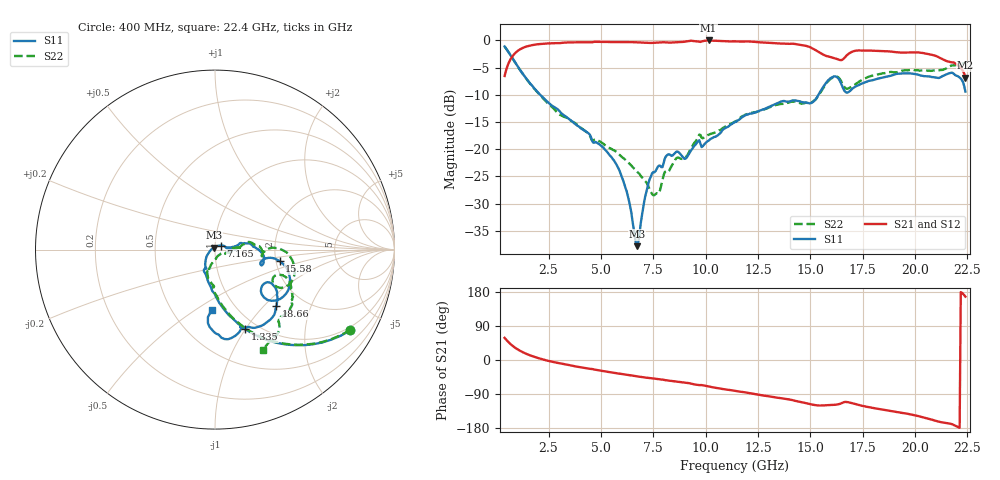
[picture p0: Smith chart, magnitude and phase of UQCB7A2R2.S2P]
!  Part Number  UQCB7A2R2	Mounting Orientation: Vertical
!  Description: RF capacitors
!  Application: Coupling, Bypass, Tuning, DC Block
!  Filters, Matching
# GHZ S DB R 50
! Freq  |S11|  S11 Ph  |S21|  S21 Ph  |S12|  S12 Ph  |S22|  S22 Ph
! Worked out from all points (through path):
!   401 points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, 400 MHz to 22.4 GHz, reference 50 ohm
!   highest |S21| = -0.03 dB at 10.13 GHz (marker M1); lowest = -6.9 dB at 22.4 GHz (marker M2)
!   group delay of S21, straight-line fit = 23.9 ps
!   lowest |S11| = -37.8 dB at 6.725 GHz (marker M3), VSWR 1.03, Z = 49.4 + j1.11 ohm
!   |S11| at or under -10 dB: 2.1 GHz to 15.38 GHz (13.28 GHz wide, 152 % of centre)
!   |S22| runs from -28.4 to -1.1 dB; largest |S21 - S12| = 0.0084
!   S11 on the Smith chart (normalised r, x): 400 MHz: 0.87, -3.42; 1.335 GHz: 0.87, -0.99; 7.165 GHz: 1.07, +0.05; 15.58 GHz: 2.09, -0.31; 18.66 GHz: 1.47, -1.19; 22.4 GHz: 0.77, -0.59
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0.4  -1.13 -30.9  -6.55 58.5  -6.58 58.5  -1.15 -30.7
1.335  -6.51 -69.2  -1.29 18.8  -1.32 18.8  -6.53 -68.7
2.27  -10.65 -85.8  -0.61 0.8  -0.63 0.9  -10.80 -85.1
4.085  -16.29 -108.4  -0.38 -19.7  -0.40 -19.6  -16.19 -104.8
5.79  -23.17 -136.4  -0.31 -35.2  -0.32 -35.1  -20.69 -105.5
6.23  -27.73 -151.8  -0.33 -39.1  -0.32 -39.0  -22.12 -102.2
6.725  -37.79 119.2  -0.38 -43.3  -0.38 -43.1  -24.10 -94.1
7.165  -27.88 34.4  -0.47 -46.5  -0.46 -46.4  -26.08 -82.8
7.77  -23.01 5.1  -0.43 -50.4  -0.42 -50.2  -28.09 -34.7
8.54  -20.67 -1.5  -0.39 -56.2  -0.37 -56.1  -21.95 -11.7
10.135  -18.43 9.7  -0.03 -69.9  -0.01 -69.8  -17.36 4.0
11.4  -15.01 11.2  -0.20 -81.5  -0.19 -81.4  -14.92 12.2
14.095  -11.12 -13.7  -0.64 -105.2  -0.61 -105.3  -11.27 -4.0
15.085  -11.43 -13.4  -1.46 -117.7  -1.44 -117.8  -11.32 -2.8
15.58  -8.74 -10.0  -2.56 -120.1  -2.56 -120.2  -8.95 1.1
16.185  -6.63 -31.6  -3.32 -118.1  -3.29 -118.2  -6.66 -18.5
16.68  -9.51 -39.6  -2.99 -110.6  -2.96 -110.8  -8.81 -28.1
18.66  -6.64 -42.6  -2.01 -132.9  -1.98 -133.0  -5.88 -31.2
18.77  -6.56 -43.7  -2.04 -134.2  -1.98 -134.2  -5.85 -32.5
20.915  -6.80 -71.0  -2.77 -159.4  -2.74 -159.7  -5.54 -46.3
21.795  -6.00 -83.9  -4.03 -170.1  -4.00 -170.4  -4.62 -55.2
22.4  -9.42 -93.2  -6.87 167.1  -6.87 166.6  -4.17 -64.3
